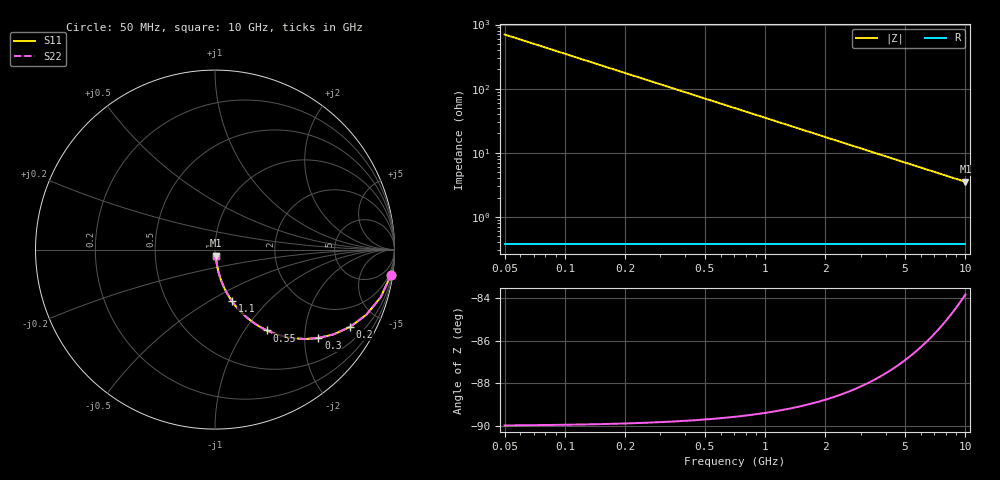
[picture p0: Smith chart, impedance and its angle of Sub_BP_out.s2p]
! Created Thu Jul 12 14:07:50 2018
# ghz S ma R 50
! 2 Port Network Data from SP1.SP block
! freq  magS11  angS11  magS21  angS21  magS12  angS12  magS22  angS22
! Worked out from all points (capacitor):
!   200 points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, 50 MHz to 10 GHz, reference 50 ohm
!   read as one part in series: C = 4.55 pF near 100 MHz
!   lowest |Z| = 3.52 ohm at 10 GHz (marker M1)
!   S11 on the Smith chart (normalised r, x): 50 MHz: 1, -14; 200 MHz: 1.01, -3.50; 300 MHz: 1.01, -2.33; 550 MHz: 1.01, -1.27; 1.1 GHz: 1.01, -0.64; 10 GHz: 1.01, -0.07
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0.05  0.9899 -8.1  0.1414 81.8  0.1414 81.8  0.9899 -8.1
0.1  0.9613 -15.9  0.2746 74.0  0.2746 74.0  0.9613 -15.9
0.15  0.9186 -23.2  0.3936 66.7  0.3936 66.7  0.9186 -23.2
0.2  0.8675 -29.7  0.4956 60.2  0.4956 60.2  0.8675 -29.7
0.25  0.8127 -35.5  0.5804 54.4  0.5804 54.4  0.8127 -35.5
0.3  0.7581 -40.5  0.6497 49.3  0.6497 49.3  0.7581 -40.5
0.4  0.6572 -48.7  0.7509 41.1  0.7509 41.1  0.6572 -48.7
0.45  0.6126 -51.9  0.7875 37.8  0.7875 37.8  0.6126 -51.9
0.55  0.5355 -57.3  0.8414 32.4  0.8414 32.4  0.5355 -57.3
0.65  0.4728 -61.4  0.8779 28.2  0.8779 28.2  0.4728 -61.4
0.8  0.3996 -66.0  0.9132 23.6  0.9132 23.6  0.3996 -66.0
0.95  0.3446 -69.3  0.9352 20.2  0.9352 20.2  0.3446 -69.3
1.1  0.3022 -71.7  0.9497 17.6  0.9497 17.6  0.3022 -71.7
1.4  0.2417 -75.1  0.9667 14.0  0.9667 14.0  0.2417 -75.1
1.75  0.1955 -77.6  0.977 11.3  0.977 11.3  0.1955 -77.6
2.5  0.1382 -80.5  0.9867 7.9  0.9867 7.9  0.1382 -80.5
3.4  0.1021 -82.0  0.991 5.9  0.991 5.9  0.1021 -82.0
4.15  0.08382 -82.6  0.9927 4.8  0.9927 4.8  0.08382 -82.6
5.05  0.06899 -82.9  0.9939 4.0  0.9939 4.0  0.06899 -82.9
6.7  0.05211 -82.9  0.9949 3.0  0.9949 3.0  0.05211 -82.9
8.35  0.0419 -82.5  0.9954 2.4  0.9954 2.4  0.0419 -82.5
10  0.03505 -81.8  0.9956 2.0  0.9956 2.0  0.03505 -81.8
